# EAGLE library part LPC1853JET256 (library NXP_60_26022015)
32-bit ARM Cortex-M3 MCU; up to 1 MB flash and 136 kB SRAM; Ethernet, two High-speed USB, LCD, EMC The LPC185x/3x/2x/1x are ARM Cortex-M3 based microcontrollers for embedded applications. The ARM Cortex-M3 is a next generation core that offers system enhancements such as low power consumption, enhanced debug features, and a high level of support block integration. The LPC185x/3x/2x/1x operate at CPU frequencies of up to 180 MHz. The ARM Cortex-M3 CPU incorporates a 3-stage pipeline and uses a Harvard architecture with separate local instruction and data buses as well as a third bus for peripherals. The ARM Cortex-M3 CPU also includes an internal prefetch unit that supports speculative branching. The LPC185x/3x/2x/1x include up to 1 MB of flash and 136 kB of on-chip SRAM, 16 kB of EEPROM memory, a quad SPI Flash Interface (SPIFI), a State Configurable Timer (SCT) subsystem, two High-speed USB controllers, Ethernet, LCD, an external memory controller, and multiple digital and analog peripherals. AAL Eindhoven MK
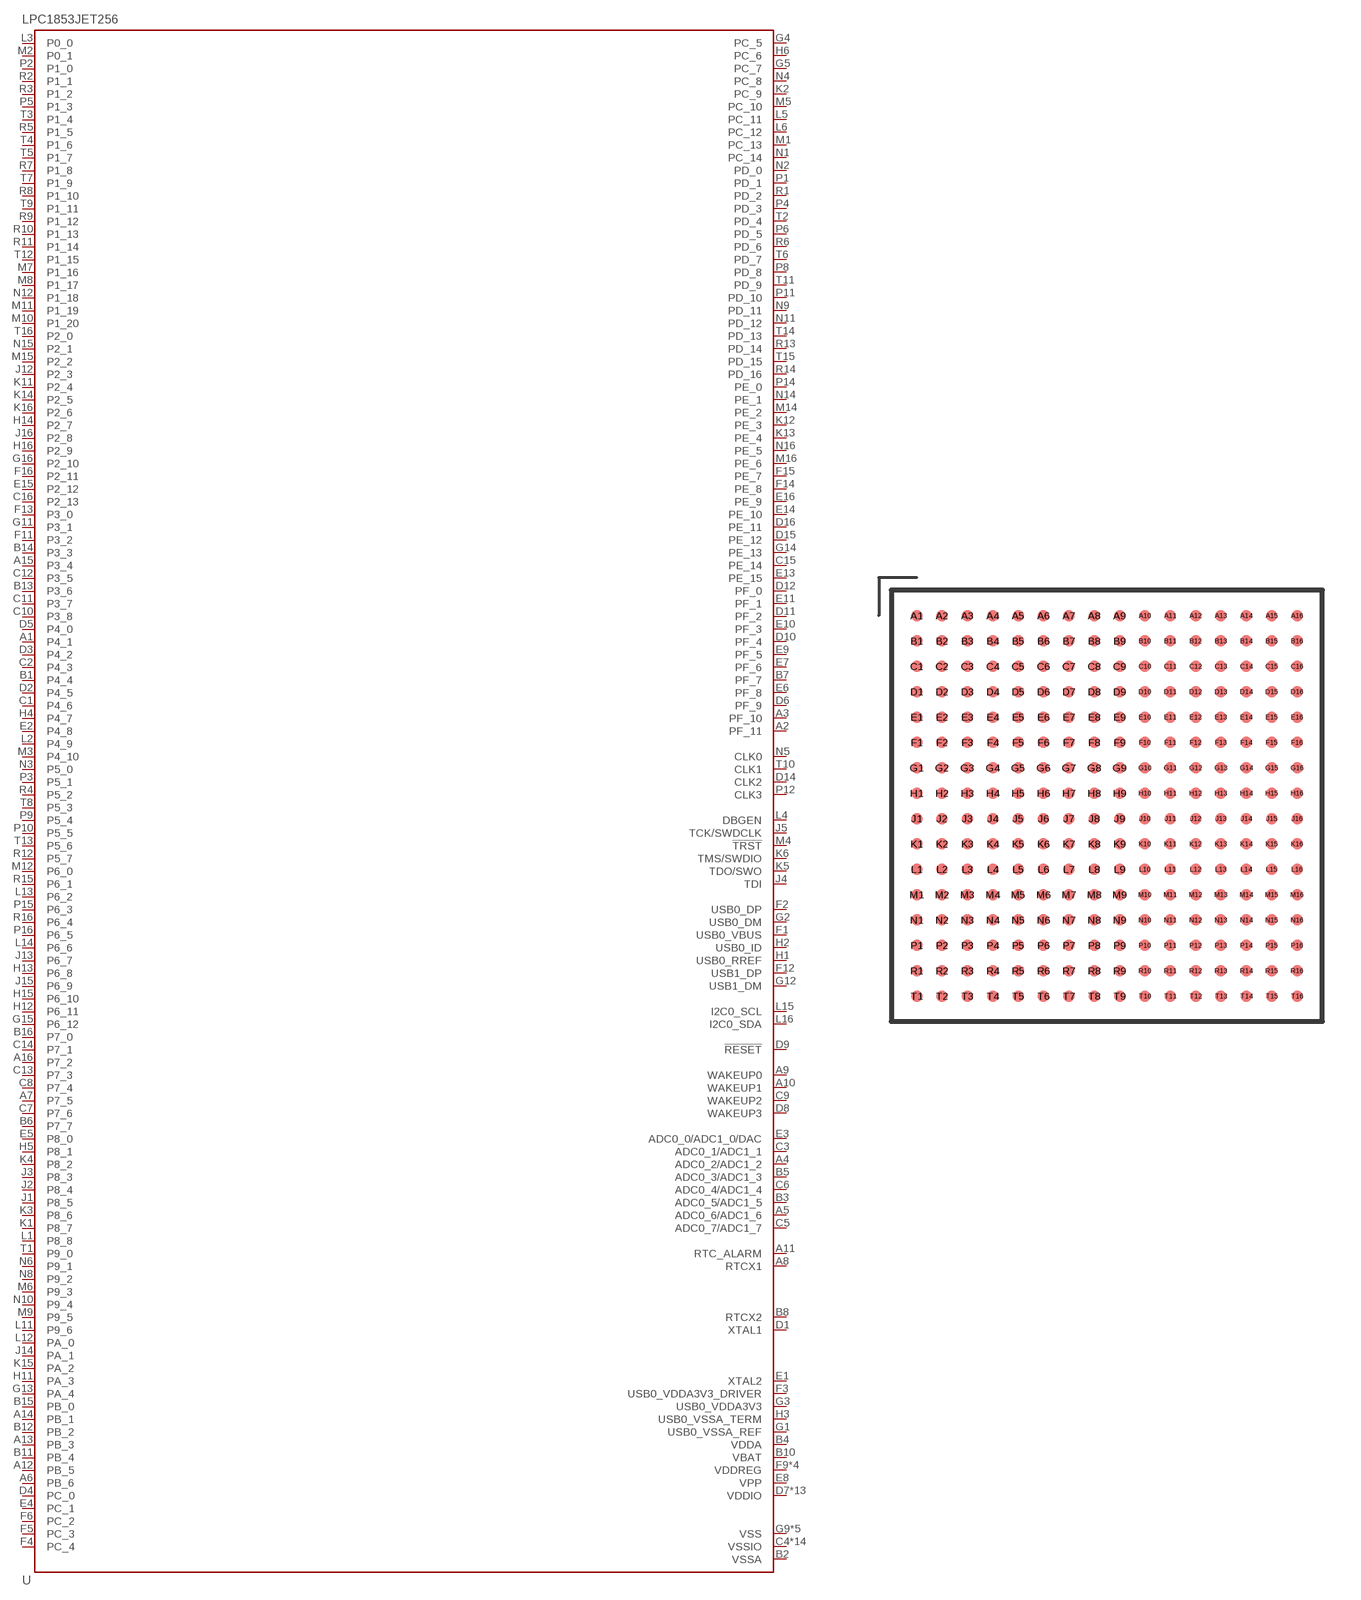
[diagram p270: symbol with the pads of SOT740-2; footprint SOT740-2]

Designator prefix U

## LPC1853JET256 (ADC: 8; ETHERNET: yes; FLASH: 512kB; GPIO: 164; LCD: yes; PWM: yes; QEI: yes; SRAM: 136kB; TEMPERATURE_RANGE: -40 °C to +105 °C; USB0: Host/OTG; USB1: Host/ULPI)  [SOT740-2]
A1  P4_1
A2  PF_11
A3  PF_10
A4  ADC0_2/ADC1_2
A5  ADC0_6/ADC1_6
A6  PB_6
A7  P7_5
A8  RTCX1
A9  WAKEUP0
A10  WAKEUP1
A11  RTC_ALARM
A12  PB_5
A13  PB_3
A14  PB_1
A15  P3_4
A16  P7_2
B1  P4_4
B2  VSSA
B3  ADC0_5/ADC1_5
B4  VDDA
B5  ADC0_3/ADC1_3
B6  P7_7
B7  PF_7
B8  RTCX2
B10  VBAT
B11  PB_4
B12  PB_2
B13  P3_6
B14  P3_3
B15  PB_0
B16  P7_0
C1  P4_6
C2  P4_3
C3  ADC0_1/ADC1_1
C4  VSSIO
C5  ADC0_7/ADC1_7
C6  ADC0_4/ADC1_4
C7  P7_6
C8  P7_4
C9  WAKEUP2
C10  P3_8
C11  P3_7
C12  P3_5
C13  P7_3
C14  P7_1
C15  PE_14
C16  P2_13
D1  XTAL1
D2  P4_5
D3  P4_2
D4  PC_0
D5  P4_0
D6  PF_9
D7  VDDIO
D8  WAKEUP3
D9  !RESET!
D10  PF_4
D11  PF_2
D12  PF_0
D13  VSSIO
D14  CLK2
D15  PE_12
D16  PE_11
E1  XTAL2
E2  P4_8
E3  ADC0_0/ADC1_0/DAC
E4  PC_1
E5  P8_0
E6  PF_8
E7  PF_6
E8  VPP
E9  PF_5
E10  PF_3
E11  PF_1
E12  VDDIO
E13  PE_15
E14  PE_10
E15  P2_12
E16  PE_9
F1  USB0_VBUS
F2  USB0_DP
F3  USB0_VDDA3V3_DRIVER
F4  PC_4
F5  PC_3
F6  PC_2
F7  VDDIO
F8  VDDIO
F9  VDDREG
F10  VDDREG
F11  P3_2
F12  USB1_DP
F13  P3_0
F14  PE_8
F15  PE_7
F16  P2_11
G1  USB0_VSSA_REF
G2  USB0_DM
G3  USB0_VDDA3V3
G4  PC_5
G5  PC_7
G6  VSSIO
G7  VSSIO
G8  VSSIO
G9  VSS
G10  VDDIO
G11  P3_1
G12  USB1_DM
G13  PA_4
G14  PE_13
G15  P6_12
G16  P2_10
H1  USB0_RREF
H2  USB0_ID
H3  USB0_VSSA_TERM
H4  P4_7
H5  P8_1
H6  PC_6
H7  VSS
H8  VSSIO
H9  VSSIO
H10  VDDIO
H11  PA_3
H12  P6_11
H13  P6_8
H14  P2_7
H15  P6_10
H16  P2_9
J1  P8_5
J2  P8_4
J3  P8_3
J4  TDI
J5  TCK/SWDCLK
J6  VDDIO
J7  VDDIO
J8  VSSIO
J9  VSSIO
J10  VSS
J11  VSS
J12  P2_3
J13  P6_7
J14  PA_1
J15  P6_9
J16  P2_8
K1  P8_7
K2  PC_9
K3  P8_6
K4  P8_2
K5  TDO/SWO
K6  TMS/SWDIO
K7  VDDIO
K8  VSS
K9  VSSIO
K10  VSSIO
K11  P2_4
K12  PE_3
K13  PE_4
K14  P2_5
K15  PA_2
K16  P2_6
L1  P8_8
L2  P4_9
L3  P0_0
L4  DBGEN
L5  PC_11
L6  PC_12
L7  VDDREG
L8  VDDREG
L9  VDDIO
L10  VDDIO
L11  P9_6
L12  PA_0
L13  P6_2
L14  P6_6
L15  I2C0_SCL
L16  I2C0_SDA
M1  PC_13
M2  P0_1
M3  P4_10
M4  !TRST!
M5  PC_10
M6  P9_3
M7  P1_16
M8  P1_17
M9  P9_5
M10  P1_20
M11  P1_19
M12  P6_0
M13  VSSIO
M14  PE_2
M15  P2_2
M16  PE_6
N1  PC_14
N2  PD_0
N3  P5_0
N4  PC_8
N5  CLK0
N6  P9_1
N7  VDDIO
N8  P9_2
N9  PD_11
N10  P9_4
N11  PD_12
N12  P1_18
N13  VDDIO
N14  PE_1
N15  P2_1
N16  PE_5
P1  PD_1
P2  P1_0
P3  P5_1
P4  PD_3
P5  P1_3
P6  PD_5
P7  VSSIO
P8  PD_8
P9  P5_4
P10  P5_5
P11  PD_10
P12  CLK3
P13  VSSIO
P14  PE_0
P15  P6_3
P16  P6_5
R1  PD_2
R2  P1_1
R3  P1_2
R4  P5_2
R5  P1_5
R6  PD_6
R7  P1_8
R8  P1_10
R9  P1_12
R10  P1_13
R11  P1_14
R12  P5_7
R13  PD_14
R14  PD_16
R15  P6_1
R16  P6_4
T1  P9_0
T2  PD_4
T3  P1_4
T4  P1_6
T5  P1_7
T6  PD_7
T7  P1_9
T8  P5_3
T9  P1_11
T10  CLK1
T11  PD_9
T12  P1_15
T13  P5_6
T14  PD_13
T15  PD_15
T16  P2_0

## Footprint SOT740-2 (pad centres in mm)
SOT740-2 LBGA256: plastic low profile ball grid array package; 256 balls; body 17 x 17 x 1 mm JEDEC: MO-192 IEC: -- JEITA: --
smd 0.45 x 0.45: A1 -7.5,7.5; A2 -6.5,7.5; A3 -5.5,7.5; A4 -4.5,7.5; A5 -3.5,7.5; A6 -2.5,7.5; A7 -1.5,7.5; A8 -0.5,7.5; A9 0.5,7.5; A10 1.5,7.5; A11 2.5,7.5; A12 3.5,7.5; A13 4.5,7.5; A14 5.5,7.5; A15 6.5,7.5; A16 7.5,7.5; B1 -7.5,6.5; B2 -6.5,6.5; B3 -5.5,6.5; B4 -4.5,6.5; B5 -3.5,6.5; B6 -2.5,6.5; B7 -1.5,6.5; B8 -0.5,6.5; B9 0.5,6.5; B10 1.5,6.5; B11 2.5,6.5; B12 3.5,6.5; B13 4.5,6.5; B14 5.5,6.5; B15 6.5,6.5; B16 7.5,6.5; C1 -7.5,5.5; C2 -6.5,5.5; C3 -5.5,5.5; C4 -4.5,5.5; C5 -3.5,5.5; C6 -2.5,5.5; C7 -1.5,5.5; C8 -0.5,5.5; C9 0.5,5.5; C10 1.5,5.5; C11 2.5,5.5; C12 3.5,5.5; C13 4.5,5.5; C14 5.5,5.5; C15 6.5,5.5; C16 7.5,5.5; D1 -7.5,4.5; D2 -6.5,4.5; D3 -5.5,4.5; D4 -4.5,4.5; D5 -3.5,4.5; D6 -2.5,4.5; D7 -1.5,4.5; D8 -0.5,4.5; D9 0.5,4.5; D10 1.5,4.5; D11 2.5,4.5; D12 3.5,4.5; D13 4.5,4.5; D14 5.5,4.5; D15 6.5,4.5; D16 7.5,4.5; E1 -7.5,3.5; E2 -6.5,3.5; E3 -5.5,3.5; E4 -4.5,3.5; E5 -3.5,3.5; E6 -2.5,3.5; E7 -1.5,3.5; E8 -0.5,3.5; E9 0.5,3.5; E10 1.5,3.5; E11 2.5,3.5; E12 3.5,3.5; E13 4.5,3.5; E14 5.5,3.5; E15 6.5,3.5; E16 7.5,3.5; F1 -7.5,2.5; F2 -6.5,2.5; F3 -5.5,2.5; F4 -4.5,2.5; F5 -3.5,2.5; F6 -2.5,2.5; F7 -1.5,2.5; F8 -0.5,2.5; F9 0.5,2.5; F10 1.5,2.5; F11 2.5,2.5; F12 3.5,2.5; F13 4.5,2.5; F14 5.5,2.5; F15 6.5,2.5; F16 7.5,2.5; G1 -7.5,1.5; G2 -6.5,1.5; G3 -5.5,1.5; G4 -4.5,1.5; G5 -3.5,1.5; G6 -2.5,1.5; G7 -1.5,1.5; G8 -0.5,1.5; G9 0.5,1.5; G10 1.5,1.5; G11 2.5,1.5; G12 3.5,1.5; G13 4.5,1.5; G14 5.5,1.5; G15 6.5,1.5; G16 7.5,1.5; H1 -7.5,0.5; H2 -6.5,0.5; H3 -5.5,0.5; H4 -4.5,0.5; H5 -3.5,0.5; H6 -2.5,0.5; H7 -1.5,0.5; H8 -0.5,0.5; H9 0.5,0.5; H10 1.5,0.5; H11 2.5,0.5; H12 3.5,0.5; H13 4.5,0.5; H14 5.5,0.5; H15 6.5,0.5; H16 7.5,0.5; J1 -7.5,-0.5; J2 -6.5,-0.5; J3 -5.5,-0.5; J4 -4.5,-0.5; J5 -3.5,-0.5; J6 -2.5,-0.5; J7 -1.5,-0.5; J8 -0.5,-0.5; J9 0.5,-0.5; J10 1.5,-0.5; J11 2.5,-0.5; J12 3.5,-0.5; J13 4.5,-0.5; J14 5.5,-0.5; J15 6.5,-0.5; J16 7.5,-0.5; K1 -7.5,-1.5; K2 -6.5,-1.5; K3 -5.5,-1.5; K4 -4.5,-1.5; K5 -3.5,-1.5; K6 -2.5,-1.5; K7 -1.5,-1.5; K8 -0.5,-1.5; K9 0.5,-1.5; K10 1.5,-1.5; K11 2.5,-1.5; K12 3.5,-1.5; K13 4.5,-1.5; K14 5.5,-1.5; K15 6.5,-1.5; K16 7.5,-1.5; L1 -7.5,-2.5; L2 -6.5,-2.5; L3 -5.5,-2.5; L4 -4.5,-2.5; L5 -3.5,-2.5; L6 -2.5,-2.5; L7 -1.5,-2.5; L8 -0.5,-2.5; L9 0.5,-2.5; L10 1.5,-2.5; L11 2.5,-2.5; L12 3.5,-2.5; L13 4.5,-2.5; L14 5.5,-2.5; L15 6.5,-2.5; L16 7.5,-2.5; M1 -7.5,-3.5; M2 -6.5,-3.5; M3 -5.5,-3.5; M4 -4.5,-3.5; M5 -3.5,-3.5; M6 -2.5,-3.5; M7 -1.5,-3.5; M8 -0.5,-3.5; M9 0.5,-3.5; M10 1.5,-3.5; M11 2.5,-3.5; M12 3.5,-3.5; M13 4.5,-3.5; M14 5.5,-3.5; M15 6.5,-3.5; M16 7.5,-3.5; N1 -7.5,-4.5; N2 -6.5,-4.5; N3 -5.5,-4.5; N4 -4.5,-4.5; N5 -3.5,-4.5; N6 -2.5,-4.5; N7 -1.5,-4.5; N8 -0.5,-4.5; N9 0.5,-4.5; N10 1.5,-4.5; N11 2.5,-4.5; N12 3.5,-4.5; N13 4.5,-4.5; N14 5.5,-4.5; N15 6.5,-4.5; N16 7.5,-4.5; P1 -7.5,-5.5; P2 -6.5,-5.5; P3 -5.5,-5.5; P4 -4.5,-5.5; P5 -3.5,-5.5; P6 -2.5,-5.5; P7 -1.5,-5.5; P8 -0.5,-5.5; P9 0.5,-5.5; P10 1.5,-5.5; P11 2.5,-5.5; P12 3.5,-5.5; P13 4.5,-5.5; P14 5.5,-5.5; P15 6.5,-5.5; P16 7.5,-5.5; R1 -7.5,-6.5; R2 -6.5,-6.5; R3 -5.5,-6.5; R4 -4.5,-6.5; R5 -3.5,-6.5; R6 -2.5,-6.5; R7 -1.5,-6.5; R8 -0.5,-6.5; R9 0.5,-6.5; R10 1.5,-6.5; R11 2.5,-6.5; R12 3.5,-6.5; R13 4.5,-6.5; R14 5.5,-6.5; R15 6.5,-6.5; R16 7.5,-6.5; T1 -7.5,-7.5; T2 -6.5,-7.5; T3 -5.5,-7.5; T4 -4.5,-7.5; T5 -3.5,-7.5; T6 -2.5,-7.5; T7 -1.5,-7.5; T8 -0.5,-7.5; T9 0.5,-7.5; T10 1.5,-7.5; T11 2.5,-7.5; T12 3.5,-7.5; T13 4.5,-7.5; T14 5.5,-7.5; T15 6.5,-7.5; T16 7.5,-7.5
